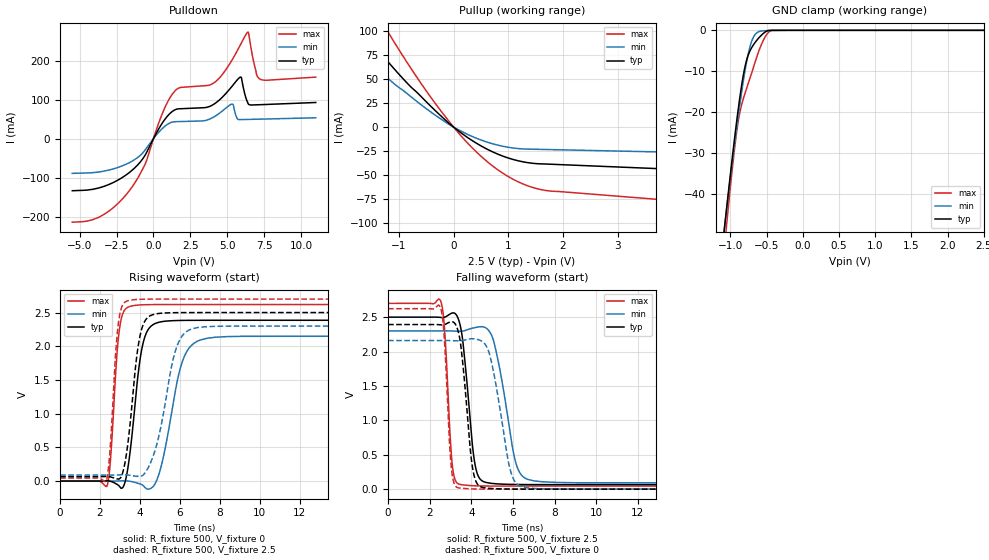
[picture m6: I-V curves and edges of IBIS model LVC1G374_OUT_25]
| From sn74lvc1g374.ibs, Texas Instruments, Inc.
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[Model]   LVC1G374_OUT_25
Model_type  3-state
Enable   Active-Low
Vref =   0
Rref =   500
Cref =   30p
Vmeas =   1.25
| variable   typ   min   max
C_comp   5.47pF   4.63pF   6.47pF
| C_pullup   8.02pF   5.55pF   9.05pF
| C_pulldown   8.86pF   6.15pF   13.06pF
| C_tri-state   5.47pF   4.63pF   6.47pF
[Temperature Range]   40   100   -40
| Ambient temperature   25   85   -40
[Voltage range]   2.5   2.3   2.7
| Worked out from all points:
|   slope of the pulldown table from 0 to 0.375 V, typ, clamps not added: 14.3 ohm
|   slope of the pullup table from 0 to 0.375 V, typ, clamps not added: 24.6 ohm
|   GND clamp passes 1 mA (typ) near -0.56 V on its own axis
|   rising waveform, R_fixture 500, V_fixture 0: 20-80 % time 538ps typ, 842ps min, 338ps max; typ from 0 V to 2.38 V
|   falling waveform, R_fixture 500, V_fixture 2.5: 20-80 % time 446ps typ, 731ps min, 276ps max; typ from 2.5 V to 0.066 V
|   rising waveform, R_fixture 500, V_fixture 2.5: 20-80 % time 526ps typ, 875ps min, 329ps max; typ from 0.066 V to 2.5 V
|   falling waveform, R_fixture 500, V_fixture 0: 20-80 % time 425ps typ, 707ps min, 262ps max; typ from 2.39 V to 0 V
[GND Clamp]
| LVC1G374_OUT_25
|   Voltage   I(typ)   I(min)   I(max)
-5.5V     -897.8mA   -832.4mA   -1.016A
-1.085V   -48.68mA   -48.61mA   -53.3mA
-1.055V   -43.78mA   -44.08mA   -47.81mA
-960mV    -28.9mA    -30.22mA   -31.49mA
-910mV    -21.66mA   -23.34mA   -24.31mA
-860mV    -15.14mA   -16.88mA   -19.23mA
-795mV    -8.582mA   -9.485mA   -15.18mA
-730mV    -5.007mA   -3.989mA   -11.68mA
-680mV    -3.482mA   -1.588mA   -8.92mA
-555mV    -899.1uA   -138.8uA   -2.764mA
-465mV    -17.59uA   -54.37uA   -352.7uA
2.5V      21.23pA    56.56nA    599.5pA
[Pulldown]
| LVC1G374_OUT_25
|   Voltage   I(typ)   I(min)   I(max)
-5.5V     -133.6mA   -89.06mA   -214.3mA
-3.75V    -126.9mA   -85.75mA   -202.3mA
-2.1V     -99.38mA   -69.59mA   -154.4mA
-590mV    -43.93mA   -30.52mA   -67.68mA
1.31V     70.54mA    42.72mA    115.7mA
4.115V    88.71mA    56.03mA    143.4mA
5.335V    134.6mA    88.49mA    202.1mA
5.905V    157.9mA    48.85mA    241.4mA
6.39V     92.54mA    49.21mA    272.9mA
6.98V     86.65mA    49.71mA    165.7mA
7.19V     86.94mA    49.89mA    153.3mA
11V       92.61mA    53.43mA    157.7mA
[Pullup]
| LVC1G374_OUT_25
|   Voltage   I(typ)   I(min)   I(max)
-5.5V     412.2mA    323.3mA    577.1mA
-2.255V   142.7mA    109mA      204.4mA
-2.155V   135.2mA    103.1mA    193.8mA
-1.775V   107.3mA    81.22mA    154.7mA
-1.295V   74.05mA    55.4mA     107.6mA
-1.24V    70.4mA     52.58mA    102.4mA
-365mV    18.75mA    13.57mA    26.85mA
320mV     -13.24mA   -9.199mA   -20.35mA
960mV     -31.31mA   -20.53mA   -49.99mA
1.57V     -38.1mA    -23.07mA   -64.51mA
7.48V     -51.85mA   -30.32mA   -91.87mA
11V       -60.13mA   -34.65mA   -107.9mA
[Ramp]
| LVC1G374_OUT_25
| variable   typ   min   max
dV/dt_r   1.49/5.63E-10   1.36/8.87E-10   1.62/3.54E-10
dV/dt_f   1.50/4.66E-10   1.36/7.59E-10   1.63/2.88E-10
R_load = 500
[Rising Waveform]
| LVC1G374_OUT_25
R_fixture =   500
C_fixture =   0
L_fixture =   0
V_fixture =   0
V_fixture_min = 0
V_fixture_max = 0
|   Time   V(typ)   V(min)   V(max)
0s        133.5pV    5.262nV    1.953nV
2.35ns    3.833mV    -30.65uV   -71.8mV
2.525ns   -3.22mV    -207uV     328.1mV
2.96ns    -73.59mV   2.205mV    2.224V
3.48ns    373.3mV    -2mV       2.589V
4.11ns    1.985V     -55.52mV   2.615V
4.87ns    2.349V     33.02mV    2.618V
6.075ns   2.383V     1.728V     2.619V
7.02ns    2.385V     2.092V     2.619V
24.99ns   2.385V     2.15V      2.619V
[Falling Waveform]
| LVC1G374_OUT_25
R_fixture =   500
C_fixture =   0
L_fixture =   0
V_fixture =   2.5
V_fixture_min = 2.3
V_fixture_max = 2.7
|   Time   V(typ)   V(min)   V(max)
0s        2.5V       2.3V       2.7V
2.53ns    2.495V     2.3V       2.732V
2.72ns    2.499V     2.3V       2.294V
3.075ns   2.559V     2.299V     376.8mV
3.405ns   2.447V     2.294V     72.46mV
4.145ns   415mV      2.346V     49.44mV
4.61ns    106.5mV    2.356V     46.39mV
6.135ns   68.33mV    384.2mV    44.77mV
6.705ns   66.83mV    142.6mV    44.71mV
24.99ns   65.57mV    89.97mV    44.64mV
[Rising Waveform]
| LVC1G374_OUT_25
R_fixture =   500
C_fixture =   0
L_fixture =   0
V_fixture =   2.5
V_fixture_min = 2.3
V_fixture_max = 2.7
|   Time   V(typ)   V(min)   V(max)
0s        65.53mV    89.9mV     44.61mV
2.335ns   69.04mV    89.88mV    27.2mV
2.5ns     64.02mV    89.74mV    458.8mV
2.9ns     30.51mV    91.19mV    2.295V
3.375ns   514.6mV    90.51mV    2.673V
3.98ns    2.121V     71.06mV    2.696V
4.635ns   2.468V     349.7mV    2.7V
5.78ns    2.498V     1.935V     2.7V
6.61ns    2.5V       2.259V     2.7V
24.99ns   2.5V       2.3V       2.7V
[Falling Waveform]
| LVC1G374_OUT_25
R_fixture =   500
C_fixture =   0
L_fixture =   0
V_fixture =   0
V_fixture_min = 0
V_fixture_max = 0
|   Time   V(typ)   V(min)   V(max)
0s        2.392V     2.16V      2.623V
2.515ns   2.389V     2.16V      2.64V
2.695ns   2.391V     2.16V      2.22V
3.025ns   2.432V     2.159V     360.2mV
3.32ns    2.341V     2.156V     23.79mV
4.05ns    325.1mV    2.186V     3.802mV
4.49ns    29.42mV    2.153V     1.371mV
5.875ns   1.757mV    271.4mV    137.2uV
6.41ns    763.5uV    36.41mV    87.84uV
24.99ns   32.87uV    51.19uV    21.19uV
